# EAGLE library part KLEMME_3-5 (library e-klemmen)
Klemme 3 5
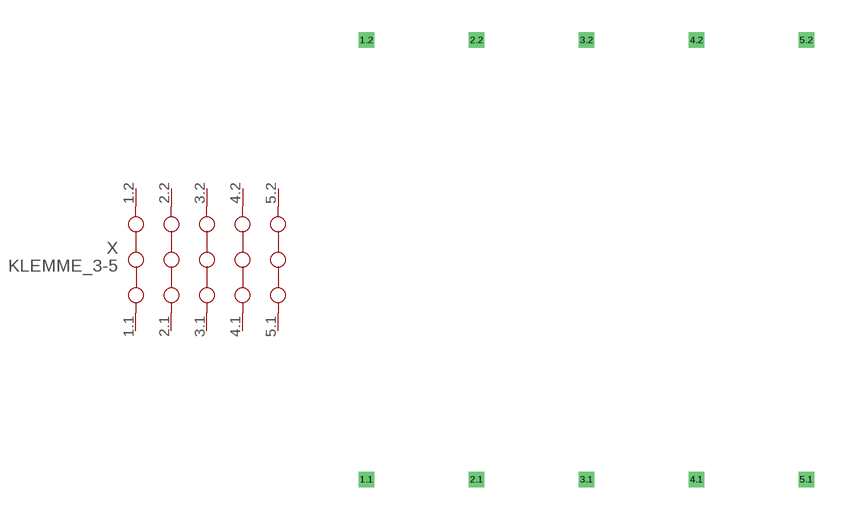
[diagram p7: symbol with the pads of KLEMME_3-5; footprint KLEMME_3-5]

Designator prefix X

## KLEMME_3-5  [KLEMME_3-5]
1.1  1.1  pas
1.2  1.2  pas
2.1  2.1  pas
2.2  2.2  pas
3.1  3.1  pas
3.2  3.2  pas
4.1  4.1  pas
4.2  4.2  pas
5.1  5.1  pas
5.2  5.2  pas

## Footprint KLEMME_3-5 (pad centres in mm)
Dummy
drill 0.2 pad 0.6 square: 1.1 0,-10.16; 1.2 0,10.16; 2.1 5.08,-10.16; 2.2 5.08,10.16; 3.1 10.16,-10.16; 3.2 10.16,10.16; 4.1 15.24,-10.16; 4.2 15.24,10.16; 5.1 20.32,-10.16; 5.2 20.32,10.16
